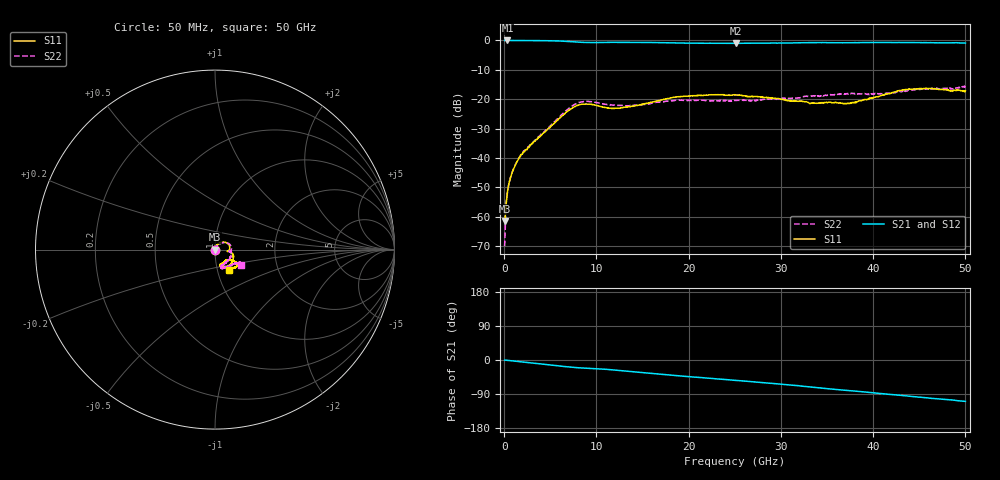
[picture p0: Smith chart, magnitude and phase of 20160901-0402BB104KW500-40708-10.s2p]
# MHZ S RI R 50
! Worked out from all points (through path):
!   801 points, 50 MHz to 50 GHz, reference 50 ohm
!   highest |S21| = 0.00 dB at 362.2 MHz (marker M1); lowest = -1.0 dB at 25.15 GHz (marker M2)
!   group delay of S21, straight-line fit = 5.92 ps
!   lowest |S11| = -61.4 dB at 50 MHz (marker M3), VSWR 1.00, Z = 49.9 + j0.0405 ohm
!   |S11| at or under -10 dB: start of sweep to end of sweep
!   |S22| runs from -70.0 to -15.4 dB; largest |S21 - S12| = 0.013
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50  -0.000752 0.000406  1 -0.00191  1 -0.00303  -0.00026 0.000183
362.188  0.00042 0.00266  1 -0.017  0.999 -0.017  0.000455 0.00262
424.625  0.00058 0.00303  0.999 -0.019  0.999 -0.02  0.000598 0.00303
549.5  0.000818 0.0038  0.999 -0.025  0.999 -0.025  0.000945 0.00375
861.688  0.00148 0.0055  0.998 -0.038  0.998 -0.039  0.00164 0.00544
1298.75  0.00218 0.00781  0.996 -0.058  0.996 -0.058  0.00267 0.00777
1923.125  0.00381 0.011  0.993 -0.085  0.993 -0.086  0.00484 0.011
6543.5  0.039 0.041  0.926 -0.288  0.926 -0.289  0.047 0.039
7604.938  0.064 0.038  0.891 -0.321  0.891 -0.322  0.073 0.036
8416.625  0.079 0.024  0.868 -0.333  0.867 -0.334  0.088 0.021
12287.75  0.07 -0.00784  0.827 -0.425  0.827 -0.426  0.078 -0.011
14535.5  0.079 -0.01  0.785 -0.497  0.785 -0.498  0.079 -0.00983
16720.81  0.093 -0.019  0.731 -0.557  0.73 -0.558  0.088 -0.014
19655.38  0.101 -0.051  0.657 -0.618  0.657 -0.619  0.088 -0.039
25025  0.068 -0.097  0.53 -0.72  0.529 -0.721  0.053 -0.08
25149.88  0.066 -0.098  0.526 -0.722  0.525 -0.723  0.052 -0.08
33391.62  0.034 -0.08  0.29 -0.873  0.288 -0.874  0.045 -0.105
37325.19  0.062 -0.057  0.15 -0.902  0.146 -0.904  0.065 -0.105
41695.81  0.105 -0.065  -0.00996 -0.924  -0.013 -0.927  0.095 -0.084
45192.31  0.126 -0.086  -0.134 -0.91  -0.139 -0.909  0.13 -0.078
48626.38  0.094 -0.099  -0.244 -0.881  -0.249 -0.876  0.131 -0.075
50000  0.076 -0.116  -0.297 -0.854  -0.299 -0.853  0.147 -0.084
